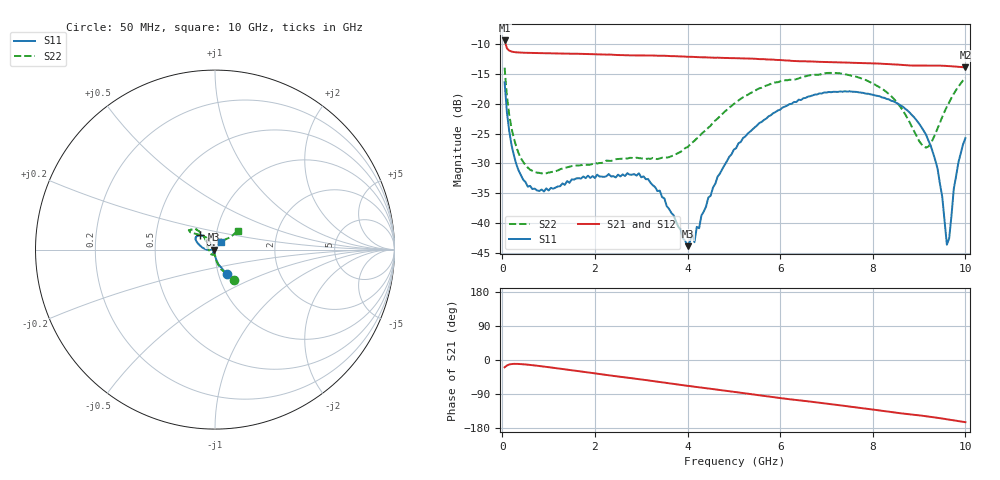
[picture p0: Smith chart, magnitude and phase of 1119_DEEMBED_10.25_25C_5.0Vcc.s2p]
!Hittite Microwave Corp.
!Digital Attenuator/PhaseShifter Rev 1.4.0
!Filename: C:\DATA\DATA\1119_DEEMBED_10.25_25C_5.0Vcc.s2p
!VNA ID: Agilent Technologies,N5224A,MY51441122,A.10.45.03
!Device type:
!2 Port Calibration.
!Temp(C): 25
!Lot Number:
!Serial Number:
!Operator:
!Misc:
!Attenuator:  10.250
# GHZ S DB R 50.0
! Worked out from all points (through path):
!   200 points, 50 MHz to 10 GHz, reference 50 ohm
!   highest |S21| = -9.37 dB at 50 MHz (marker M1); lowest = -13.9 dB at 10 GHz (marker M2)
!   group delay of S21, straight-line fit = 43.9 ps
!   lowest |S11| = -43.9 dB at 4 GHz (marker M3), VSWR 1.01, Z = 49.4 - j0.0799 ohm
!   |S11| at or under -10 dB: start of sweep to end of sweep
!   |S22| runs from -31.7 to -13.9 dB; largest |S21 - S12| = 0.00088
!   S11 on the Smith chart (normalised r, x): 50 MHz: 1.10, -0.31; 6.6 GHz: 0.84, +0.14; 10 GHz: 1.06, +0.08
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0.05  -16.40 -64.4  -9.37 -19.2  -9.37 -19.2  -13.94 -57.5
0.1  -21.46 -76.8  -10.69 -14.5  -10.69 -14.5  -18.70 -72.5
0.2  -26.95 -85.5  -11.23 -10.7  -11.24 -10.7  -24.12 -83.2
0.55  -33.91 -96.4  -11.45 -12.4  -11.45 -12.4  -30.71 -93.5
1.75  -32.21 -114.0  -11.63 -31.1  -11.63 -31.1  -30.24 -110.8
2.95  -31.67 -110.0  -11.88 -50.5  -11.89 -50.6  -29.13 -148.2
3.4  -34.59 -118.4  -11.93 -58.0  -11.94 -58.0  -29.17 -169.2
4  -43.91 -172.7  -12.11 -68.0  -12.12 -68.1  -27.28 158.0
4.1  -41.80 161.2  -12.12 -69.7  -12.13 -69.8  -26.53 153.4
4.15  -43.25 154.0  -12.14 -70.5  -12.15 -70.6  -26.21 150.7
4.65  -32.22 118.7  -12.26 -78.4  -12.29 -78.4  -22.48 134.3
5.05  -27.45 120.0  -12.35 -84.7  -12.37 -84.8  -19.74 129.7
6.6  -18.81 136.0  -12.89 -109.1  -12.91 -109.1  -15.30 139.7
6.7  -18.59 137.3  -12.91 -110.6  -12.92 -110.6  -15.15 140.1
8.35  -19.27 157.7  -13.33 -136.5  -13.33 -136.5  -18.37 136.2
9.05  -23.91 173.6  -13.59 -146.8  -13.59 -146.8  -26.79 101.1
9.25  -27.02 180.0  -13.58 -150.0  -13.60 -150.0  -26.67 70.5
9.5  -35.60 176.3  -13.61 -154.5  -13.62 -154.5  -22.21 45.0
9.6  -43.66 138.4  -13.66 -156.4  -13.66 -156.4  -20.50 41.4
9.65  -42.59 79.9  -13.68 -157.3  -13.69 -157.3  -19.74 40.2
9.75  -34.25 52.0  -13.73 -159.3  -13.74 -159.3  -18.30 39.1
10  -25.77 50.6  -13.91 -164.1  -13.91 -164.1  -15.62 39.7
